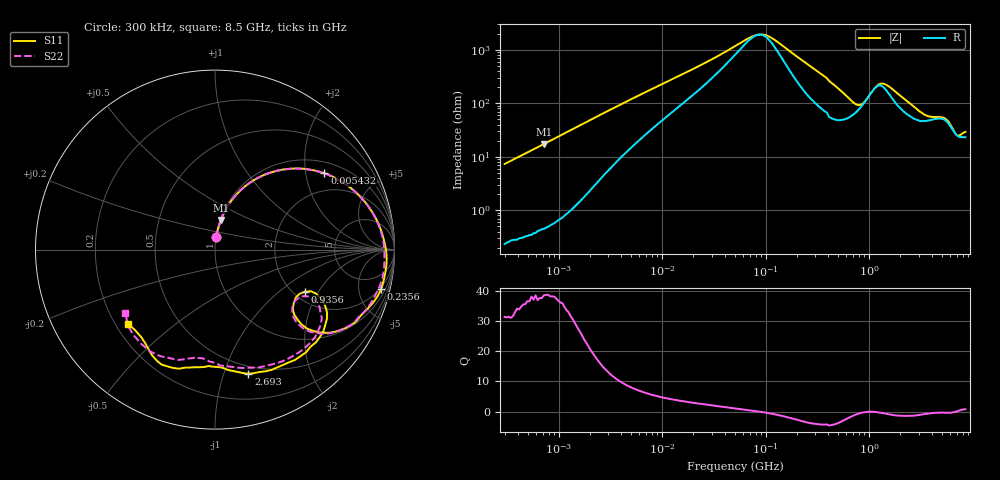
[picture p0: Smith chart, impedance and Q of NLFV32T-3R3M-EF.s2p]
! S-parameter Generated by TDK Corporation
! Copyright(C) 2015 TDK Corporation.
! All Rights Reserved.
! TDK P/N: NLFV32T-3R3M-EF (Inductors)
! Property: L=3.3uH at 7.96MHz
! Size(LxWxT): 3.2x2.5x2.2mm, 0.126x0.098x0.087inches
! Model Type: s2p (Touchstone File Format Version 1.0)
! Frequency: DC=Yes Start=0.3MHz Stop=8500MHz 225points Log-sweep
! Note:
! Model Generated on Jun. 23, 2015
! Hash(MD5):
! Port Assignments:
!  1 ---@@@--- 2
! Applicable Conditions:
!  Temperature = 25 degC
!  DC Bias Current = 0 A
!  Small Signal Operation
! Terms and conditions regarding TDK Simulation Models
! (1)This simulation model is being provided solely for informational purposes. Please refer to the specifications of the products in terms of detailed characteristics of such products.
! (2)In no event shall TDK Corporation of any of its subsidiaries be liable for any loss or damage arising, directly or indirectly,
!  From any information contained in this simulation model, including, but not limited to loss or damages arising from any inaccuracies, omissions or errors in connection with such information.
! (3)Any and all copyrights on this simulation model are owned by TDK Corporation.
!  Duplication or redistribution of this simulation model without prior written permission from TDK Corporation is prohibited.
! (4)This simulation model is subject to any modification or change without any prior notice.
! (5)Neither TDK Corporation nor any of its subsidiaries shall make any warranty, express or implied,
!  Including but not limited to the correctness, implied warranties of merchantability and fitness for a particular purpose with respect to this simulation models.
! (6)The use of this simulation model shall be deemed to have consented to the terms and conditions hereof.
# MHz S MA R 50
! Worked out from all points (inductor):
!   224 points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, 300 kHz to 8.5 GHz, reference 50 ohm
!   read as one part in series: L = 3.87 uH near 314.1 kHz
!   highest Q = 38.4 at 718.6 kHz (marker M1), where L = 3.83 uH
!   self-resonance near 85.69 MHz
!   S11 on the Smith chart (normalised r, x): 300 kHz: 1.00, +0.14; 5.432 MHz: 1.34, +2.55; 235.6 MHz: 1.81, -8.26; 935.6 MHz: 2.28, -1.54; 2.693 GHz: 0.43, -1.21; 8.5 GHz: 0.25, -0.35
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0.3  0.07098 84.2  0.9931 -4.1  0.9968 -4.5  0.07068 84.4
0.7185633  0.1678 78.8  0.9811 -9.7  0.9827 -10.0  0.1677 78.8
1.72111  0.3766 65.5  0.9113 -22.1  0.9127 -22.5  0.3769 65.5
3.12867  0.5792 50.2  0.7713 -35.3  0.7721 -35.7  0.5797 50.1
5.431819  0.7434 34.9  0.5788 -47.5  0.5792 -47.9  0.7437 34.8
9.430415  0.846 22.3  0.3909 -56.1  0.3912 -56.5  0.8463 22.2
51.67171  0.9457 2.2  0.07876 -43.2  0.07881 -43.5  0.9404 1.9
78.15234  0.9542 -0.9  0.05156 -12.4  0.05159 -12.8  0.9442 -1.3
98.34885  0.9576 -2.7  0.05034 15.2  0.05036 14.9  0.9456 -3.2
235.5662  0.9511 -13.2  0.1572 60.2  0.1573 59.8  0.9356 -13.9
283.1228  0.9394 -16.6  0.1993 59.1  0.1995 58.8  0.924 -17.3
564.2308  0.7655 -37.3  0.4573 34.7  0.4572 34.4  0.7568 -38.2
743.4462  0.5698 -39.3  0.53 10.7  0.5301 10.2  0.5712 -40.5
935.5712  0.5521 -25.1  0.4513 -10.3  0.4515 -11.2  0.5567 -27.7
1232.735  0.7149 -29.2  0.293 -10.0  0.2935 -10.5  0.7067 -32.6
1551.304  0.7636 -42.7  0.3118 3.7  0.312 2.8  0.7421 -47.0
2693.286  0.7163 -74.9  0.4628 -11.3  0.4624 -12.4  0.6693 -79.4
4073.536  0.6496 -93.1  0.4767 -37.8  0.4793 -38.9  0.6094 -96.8
5126.239  0.6787 -104.3  0.428 -49.9  0.4272 -50.3  0.6348 -105.7
6161.135  0.7063 -115.0  0.4289 -55.4  0.4244 -55.7  0.6725 -122.3
7072.242  0.6702 -123.2  0.4607 -65.4  0.4626 -66.2  0.6449 -138.6
8500  0.6361 -139.5  0.4167 -91.7  0.4156 -90.9  0.6127 -145.1
